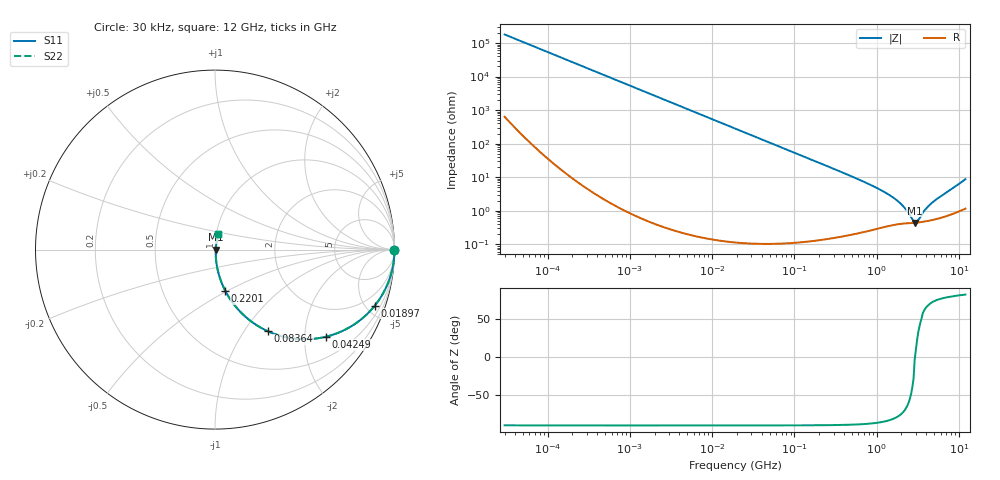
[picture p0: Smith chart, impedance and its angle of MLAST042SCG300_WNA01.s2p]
! MLAST042SCG300_WNA01  S-PARAMETER MODEL  ( General Type )
! Model Generated by TAIYO YUDEN Corporation (http://www.ty-top.com)
! Version 1.0
! TAIYO YUDEN Control No. 150820
! Copyright(c) 2015 TAIYO YUDEN CO.,LTD. All Rights Reserved.
! Product Description (link to TY-COMPAS)
! https://ds.yuden.co.jp/TYCOMPAS/or/detail?pn=MLAST042SCG300JWNA01&u=M
! Products Name : Multilayer Ceramic Capacitors
! Characteristics :
!  Capacitance : 30 pF , Rated Voltage : 25V , TCC : CG / C0G
!  Case Size : 0.4 x 0.2 / 0.016 x 0.008 [mm/inch] , Thickness : 0.2 / 0.008 [mm/inch]
!  (Conditions: Temperature = 25 degC , DC Bias Current/Voltage = 0A / 0V)
! External Node Assignments :
!  1  o---| |---o  2
! GND o---------o GND
! Frequency Range : 0.03MHz  -  12000MHz  [ 401 STEP ]
# MHz S RI R 50
! Freq[MHz].  S11 Real  S11 Imag  S21 Real  S21 Imag  S12 Real  S12 Imag  S22 Real  S22 Imag
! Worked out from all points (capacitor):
!   401 points, 30 kHz to 12 GHz, reference 50 ohm
!   read as one part in series: C = 29.5 pF near 32 kHz
!   lowest |Z| = 432 mohm at 2.904 GHz (marker M1)
!   series resonance near 2.926 GHz, so ESL is about 100 pH
!   S11 on the Smith chart (normalised r, x): 30 kHz: open; 18.97 MHz: 1.00, -5.70; 42.49 MHz: 1.00, -2.54; 83.64 MHz: 1.00, -1.29; 220.1 MHz: 1.00, -0.49; 12 GHz: 1.02, +0.17
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0.03  1 -0.000555  2.26e-06 0.000555  2.26e-06 0.000555  1 -0.000555
0.260295  1 -0.00482  2.46e-05 0.00482  2.46e-05 0.00482  1 -0.00482
2.258455  0.9982 -0.0417  0.00175 0.0417  0.00175 0.0417  0.9982 -0.0417
7.211021  0.9825 -0.1311  0.0175 0.1311  0.0175 0.1311  0.9825 -0.1311
18.97367  0.8901 -0.3125  0.1099 0.3125  0.1099 0.3125  0.8901 -0.3125
27.93914  0.7889 -0.4078  0.2111 0.4078  0.2111 0.4078  0.7889 -0.4078
42.48934  0.6177 -0.4855  0.3823 0.4855  0.3823 0.4855  0.6177 -0.4855
58.65857  0.4589 -0.4977  0.5411 0.4977  0.5411 0.4977  0.4589 -0.4977
83.63502  0.2945 -0.455  0.7055 0.455  0.7055 0.455  0.2945 -0.455
115.4622  0.1798 -0.3828  0.8202 0.3828  0.8202 0.3828  0.1798 -0.3828
164.6252  0.0976 -0.2949  0.9024 0.2949  0.9024 0.2949  0.0976 -0.2949
220.0608  0.0574 -0.2299  0.9426 0.2299  0.9426 0.2299  0.0574 -0.2299
725.66  0.00721 -0.0694  0.9928 0.0694  0.9928 0.0694  0.00721 -0.0694
1428.372  0.00438 -0.029  0.9956 0.029  0.9956 0.029  0.00438 -0.029
2036.564  0.00429 -0.0142  0.9957 0.0142  0.9957 0.0142  0.00429 -0.0142
2316.96  0.00429 -0.00932  0.9957 0.00932  0.9957 0.00932  0.00429 -0.00932
2722.352  0.00429 -0.00346  0.9957 0.00346  0.9957 0.00346  0.00429 -0.00346
2903.719  0.0043 -0.000212  0.9957 0.000212  0.9957 0.000212  0.0043 -0.000212
3198.675  0.00444 0.00276  0.9956 -0.00276  0.9956 -0.00276  0.00444 0.00276
3881.513  0.00486 0.00948  0.9951 -0.00948  0.9951 -0.00948  0.00486 0.00948
4864.487  0.00563 0.0174  0.9944 -0.0174  0.9944 -0.0174  0.00563 0.0174
12000  0.0186 0.0842  0.9814 -0.0842  0.9814 -0.0842  0.0186 0.0842
